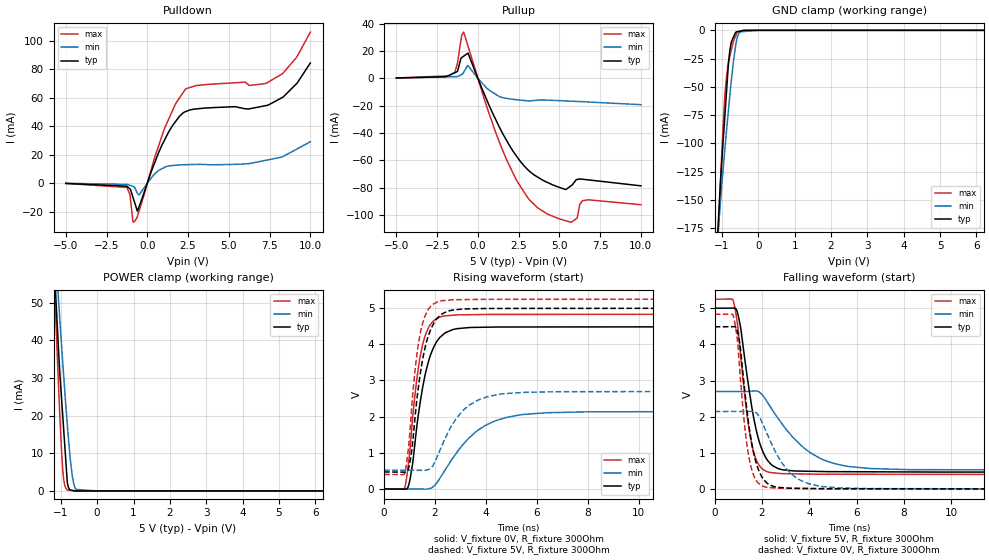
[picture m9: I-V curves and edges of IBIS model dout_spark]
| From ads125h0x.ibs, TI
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|   dout_spark Model
[Model]   dout_spark
Model_type   3-state
Polarity   Non-Inverting
Vmeas = 2.5
Vref = 0
Cref = 20pF
Rref = 100000
|   typ   min   max
C_comp   6.42159pF   5.72364pF   6.6322pF
|  Where Nom  PVT is Nominal Process,   5V,  27C
|   Fast PVT is Strong Process,   5.25V, -40C
|   Slow PVT is Weak Process,   2.7V, 135C
[Voltage Range]   5   2.7   5.25
|Junction Temperature
[Temperature Range]   27   135   -40
[Pullup Reference]   5   2.7   5.25
[Pulldown Reference]   0   0   0
[Power Clamp Reference]   5   2.7   5.25
[GND Clamp Reference]   0   0   0
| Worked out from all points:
|   slope of the pulldown table from 0 to 0.75 V, typ, clamps not added: 32.8 ohm
|   slope of the pullup table from 0 to 0.75 V, typ, clamps not added: 35 ohm
|   GND clamp passes 1 mA (typ) near -0.55 V on its own axis
|   POWER clamp passes 1 mA (typ) near -0.79 V on its own axis
|   falling waveform, V_fixture 5V, R_fixture 300Ohm: 20-80 % time 684ps typ, 1.81ns min, 515ps max; typ from 5 V to 0.47 V
|   rising waveform, V_fixture 0V, R_fixture 300Ohm: 20-80 % time 616ps typ, 1.58ns min, 474ps max; typ from 0 V to 4.49 V
|   rising waveform, V_fixture 5V, R_fixture 300Ohm: 20-80 % time 541ps typ, 1.13ns min, 424ps max; typ from 0.47 V to 5 V
|   falling waveform, V_fixture 0V, R_fixture 300Ohm: 20-80 % time 549ps typ, 1.14ns min, 431ps max; typ from 4.49 V to 0 V
[Pulldown]
|   Voltage   I(typ)   I(min)   I(max)
-5V       -193.1uA   -112.3uA   -189.6uA
-1.25V    -2.138mA   -843.3uA   -3.017mA
-1.061V   -4.07mA    -1.537mA   -8.165mA
-883.6mV  -9.75mA    -2.187mA   -26.86mA
-821.5mV  -11.96mA   -2.414mA   -27.38mA
-607.1mV  -19.61mA   -7.003mA   -23.3mA
1.02V     29.38mA    10.84mA    37.11mA
2.336V    50.09mA    12.93mA    65.81mA
7.274V    54.37mA    16.03mA    69.88mA
8.301V    60.18mA    18.51mA    76.83mA
9.175V    69.99mA    23.93mA    88.52mA
10V       84.29mA    29.04mA    105.9mA
[GND Clamp]
|   Voltage   I(typ)   I(min)   I(max)
-5V       -2.828A    -2.084A    -3.614A
-1.128V   -186.1mA   -187.3mA   -202.1mA
-1.036V   -131.3mA   -149.9mA   -130.9mA
-969.2mV  -99.24mA   -123.5mA   -84.42mA
-917.5mV  -74.58mA   -104.6mA   -56.15mA
-867.4mV  -50.7mA    -86.21mA   -38.73mA
-821.4mV  -28.77mA   -70.6mA    -28.81mA
-782.3mV  -17.58mA   -57.42mA   -22.79mA
-607.1mV  -1.389mA   -10.44mA   -3.827mA
-507.3mV  -744.4uA   -1.362mA   -1.125mA
-131.8uV  -501.4pA   0A         0A
10V       0A         0A         0A
[Pullup]
|   Voltage   I(typ)   I(min)   I(max)
-5V       265.4uA    145.6uA    281.5uA
-1.412V   4.134mA    1.221mA    4.392mA
-998.2mV  15.12mA    2.747mA    31.16mA
-881.2mV  16.12mA    4.277mA    33.83mA
-607.1mV  18.45mA    9.263mA    23.7mA
1.382V    -37.18mA   -13.67mA   -48.68mA
3.195V    -68.25mA   -16.49mA   -89.26mA
5.178V    -80.54mA   -16.42mA   -103.4mA
5.731V    -78.41mA   -16.72mA   -105.2mA
6.089V    -73.97mA   -16.91mA   -102.2mA
6.408V    -73.78mA   -17.09mA   -89.51mA
10V       -78.63mA   -19.27mA   -92.43mA
[POWER Clamp]
|   Voltage   I(typ)   I(min)   I(max)
-5V       854.4mA    670.6mA    1.098A
-1.159V   55.76mA    64.89mA    51.13mA
-1.131V   50.28mA    60.77mA    44.27mA
-1.087V   42.08mA    54.33mA    33.57mA
-1.036V   32.55mA    46.85mA    21.96mA
-952mV    20.71mA    34.84mA    6.367mA
-889.9mV  11.93mA    26.39mA    1.305mA
-821.5mV  2.266mA    17.72mA    271.4uA
-736mV    263.1uA    8.179mA    144.6uA
-684.1mV  158.4uA    3.953mA    67.61uA
-580.5mV  2.73uA     395.7uA    1.642uA
10V       0A         0A         0A
[Ramp]
R_load = 300
|   typ   min   max
dV/dt_r   2.69211/6.15679e-10   1.28754/1.57411e-09   2.89953/4.73551e-10
dV/dt_f   2.71777/6.84172e-10   1.30708/1.79649e-09   2.90858/5.13879e-10
[Falling Waveform]
V_fixture = 5V
V_fixture_min = 2.7V
V_fixture_max = 5.25V
R_fixture = 300Ohm
C_fixture = 0F
|   Time   V(typ)   V(min)   V(max)
0s        5V         2.7V       5.25V
764.9ps   5.003V     2.699V     5.24V
943.9ps   4.916V     2.699V     4.657V
1.319ns   3.367V     2.699V     2.306V
1.546ns   2.361V     2.708V     1.303V
1.836ns   1.422V     2.7V       703mV
2.179ns   849.2mV    2.451V     492.7mV
3.784ns   497.2mV    1.133V     419.3mV
5.584ns   482.7mV    634.3mV    411.7mV
20ns      470.4mV    521.2mV    402.4mV
[Rising Waveform]
V_fixture = 0V
V_fixture_min = 0V
V_fixture_max = 0V
R_fixture = 300Ohm
C_fixture = 0F
|   Time   V(typ)   V(min)   V(max)
0s        103.2uV    781.8uV    10.55uV
787.6ps   -5.114mV   706.5uV    5.199mV
943.9ps   61.91mV    691.6uV    625.4mV
1.258ns   1.565V     -1.56mV    2.885V
1.477ns   2.656V     -3.461mV   3.878V
1.789ns   3.634V     13.83mV    4.517V
2.179ns   4.181V     281.4mV    4.749V
3.584ns   4.467V     1.568V     4.82V
5.284ns   4.478V     2.042V     4.826V
20ns      4.487V     2.147V     4.833V
[Rising Waveform]
V_fixture = 5V
V_fixture_min = 2.7V
V_fixture_max = 5.25V
R_fixture = 300Ohm
C_fixture = 0F
|   Time   V(typ)   V(min)   V(max)
0s        470.4mV    521.2mV    402.4mV
787.6ps   464.6mV    517.6mV    407.2mV
943.9ps   533.7mV    516.8mV    1.064V
1.223ns   2.041V     515.5mV    3.336V
1.42ns    3.179V     514.6mV    4.303V
1.706ns   4.167V     531.7mV    4.934V
2.104ns   4.731V     923.2mV    5.176V
3.113ns   4.976V     2.177V     5.235V
4.584ns   4.991V     2.623V     5.243V
20ns      5V         2.7V       5.25V
[Falling Waveform]
|Gnd
V_fixture = 0V
V_fixture_min = 0V
V_fixture_max = 0V
R_fixture = 300Ohm
C_fixture = 0F
|   Time   V(typ)   V(min)   V(max)
0s        4.487V     2.147V     4.833V
764.9ps   4.49V      2.148V     4.823V
943.9ps   4.402V     2.148V     4.202V
1.223ns   3.011V     2.149V     2.023V
1.42ns    1.887V     2.149V     985.6mV
1.706ns   835.4mV    2.125V     294.1mV
2.034ns   297mV      1.8V       82.03mV
3.113ns   29.06mV    501.2mV    21.98mV
4.484ns   15.49mV    78.73mV    9.546mV
20ns      103.1uV    781.9uV    10.59uV
